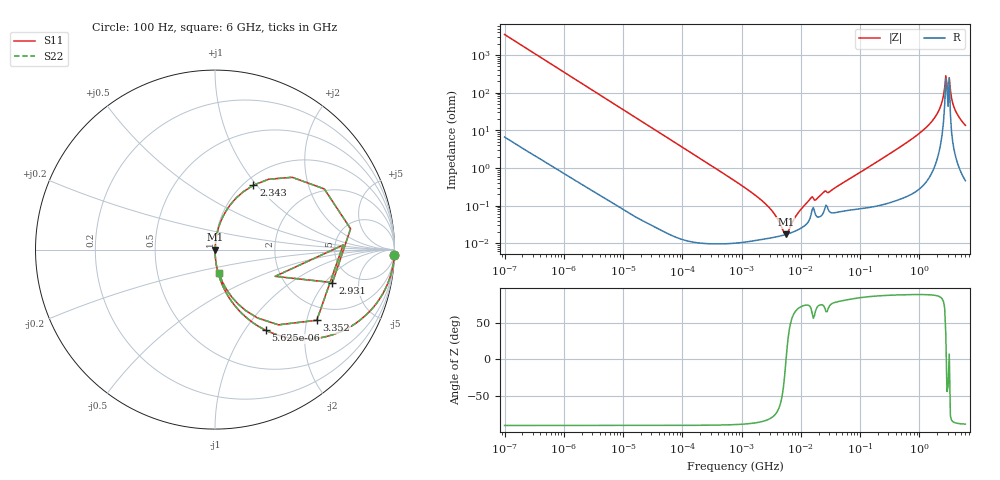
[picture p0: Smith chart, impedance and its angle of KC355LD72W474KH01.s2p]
!Murata Part Number: KC355LD72W474KH01
!These Parameters are Measured in Series Mode Connection
!Data Generated on Mar 13, 2026
!  o--ll--o
!Port1  Port2
!  o------o
!Operation Temp=25[degC], DC Bias Voltage=0[V]
!Freq. Start=100[Hz] Stop=6[GHz] 401[Steps]
# Hz S RI R 50
!Freq.(Hz) S11(Real) S11(Imag) S21(Real) S21(Imag) S12(Real) S12(Imag) S22(Real) S22(Imag)
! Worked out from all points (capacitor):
!   401 points, 100 Hz to 6 GHz, reference 50 ohm
!   read as one part in series: C = 452 nF near 109 Hz
!   lowest |Z| = 17 mohm at 5.555 MHz (marker M1)
!   series resonance near 5.638 MHz, so ESL is about 1.8 nH
!   S11 on the Smith chart (normalised r, x): 100 Hz: 1, -70; 5.625 kHz: 1.00, -1.26; 2.343 GHz: 1.11, +0.96; 2.931 GHz: 3.51, -2.40; 3.352 GHz: 1.53, -2.30; 6 GHz: 1.01, -0.27
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100  0.9991 -0.0284  0.00086 0.0284  0.00086 0.0284  0.9991 -0.0284
750  0.9564 -0.2032  0.0436 0.2032  0.0436 0.2032  0.9564 -0.2032
2008  0.7553 -0.4289  0.2447 0.4289  0.2447 0.4289  0.7553 -0.4289
5625  0.2838 -0.4498  0.7162 0.4498  0.7162 0.4498  0.2838 -0.4498
12592  0.0738 -0.2603  0.9262 0.2603  0.9262 0.2603  0.0738 -0.2603
40335  0.0079 -0.0872  0.9921 0.0872  0.9921 0.0872  0.0079 -0.0872
774597  0.00012 -0.00448  0.9999 0.00448  0.9999 0.00448  0.00012 -0.00448
2713602  0.000133 -0.000989  0.9999 0.000989  0.9999 0.000989  0.000133 -0.000989
5554849  0.000169 -1.81e-05  0.9998 1.81e-05  0.9998 1.81e-05  0.000169 -1.81e-05
9090158  0.00023 0.000609  0.9998 -0.000609  0.9998 -0.000609  0.00023 0.000609
1.555665e7  0.000781 0.00152  0.9992 -0.00152  0.9992 -0.00152  0.000781 0.00152
3.184506e7  0.000657 0.00235  0.9993 -0.00235  0.9993 -0.00235  0.000657 0.00235
3.124326e8  0.00172 0.0234  0.9983 -0.0234  0.9983 -0.0234  0.00172 0.0234
1.251881e9  0.0161 0.1096  0.9839 -0.1096  0.9839 -0.1096  0.0161 0.1096
1.95892e9  0.0752 0.2357  0.9248 -0.2357  0.9248 -0.2357  0.0752 0.2357
2.34314e9  0.2138 0.3588  0.7862 -0.3588  0.7862 -0.3588  0.2138 0.3588
2.562649e9  0.4298 0.4028  0.5702 -0.4028  0.5702 -0.4028  0.4298 0.4028
2.931063e9  0.6543 -0.1838  0.3457 0.1838  0.3457 0.1838  0.6543 -0.1838
3.352442e9  0.5671 -0.3937  0.4329 0.3937  0.4329 0.3937  0.5671 -0.3937
3.666503e9  0.2371 -0.3809  0.7629 0.3809  0.7629 0.3809  0.2371 -0.3809
4.193612e9  0.0967 -0.2678  0.9033 0.2678  0.9033 0.2678  0.0967 -0.2678
6e9  0.0223 -0.1316  0.9777 0.1316  0.9777 0.1316  0.0223 -0.1316
